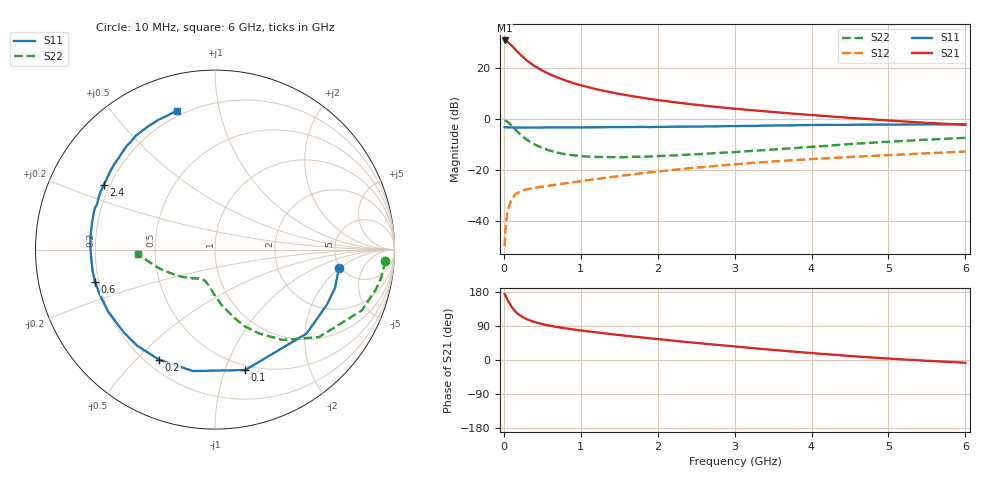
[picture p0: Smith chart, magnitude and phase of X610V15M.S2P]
! SIEMENS Small Signal Semiconductors
! BFP193W
! Si NPN RF Bipolar Junction Transistor in SOT343
! VCE = 10 V  IC = 15 mA
! Common Emitter S-Parameters:  April 1994
# GHz  S  MA  R  50
!  f  S11  S21  S12  S22
! GHz  MAG  ANG  MAG  ANG  MAG  ANG  MAG  ANG
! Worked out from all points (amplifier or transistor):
!   40 points, 10 MHz to 6 GHz, reference 50 ohm
!   highest |S21| = 31.0 dB at 10 MHz (marker M1)
!   |S21| within 3 dB of that: start of sweep to 132.5 MHz
!   unconditionally stable (mu >= 1): 1.187 GHz to 4.775 GHz
!   at 200 MHz: K = 0.28, MSG = 27.2 dB, |S12| = -28.6 dB
!   at 1.5 GHz: K = 1.07, MAG = 14.5 dB, |S12| = -22.3 dB
!   at 6 GHz: K = 0.93, MSG = 5.2 dB, |S12| = -12.7 dB
!   S11 on the Smith chart (normalised r, x): 10 MHz: 4.83, -1.92; 100 MHz: 0.46, -1.18; 200 MHz: 0.25, -0.59; 600 MHz: 0.19, -0.13; 2.4 GHz: 0.18, +0.26; 6 GHz: 0.17, +0.75
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0.01  0.698 -8.4  35.51 174.1  0.0032 77.6  0.9509 -3.8
0.02  0.7016 -17.6  35.29 170.6  0.0067 77.1  0.94 -9.4
0.03  0.6952 -26.1  34.82 166.3  0.0098 76.1  0.9242 -13.8
0.05  0.6922 -42.5  33.37 157.9  0.0157 68.8  0.8859 -22.5
0.1  0.6919 -75.9  28.39 140.7  0.0266 56.2  0.7573 -40.0
0.15  0.6877 -100.3  23.55 127.8  0.0335 47.2  0.6296 -53.1
0.2  0.6881 -116.9  19.59 119.0  0.0372 41.9  0.5286 -62.2
0.25  0.6892 -128.9  16.63 112.6  0.0402 38.9  0.4553 -69.1
0.3  0.6866 -137.5  14.28 107.5  0.0419 37.0  0.395 -74.2
0.4  0.6887 -150.0  11.12 100.1  0.0449 35.5  0.32 -82.1
0.5  0.6894 -158.7  9.079 94.7  0.0474 36.1  0.273 -87.8
0.6  0.6921 -164.8  7.633 90.4  0.0499 36.9  0.2416 -92.3
0.8  0.6908 -173.9  5.802 83.6  0.0552 39.8  0.2065 -98.8
1.1  0.6954 176.8  4.272 75.4  0.0638 43.3  0.1841 -106.4
1.3  0.6983 171.5  3.623 70.4  0.0701 45.2  0.1809 -110.3
1.6  0.7034 164.8  2.972 63.6  0.08 47.2  0.1807 -114.9
2.2  0.7141 153.3  2.186 51.1  0.1012 48.3  0.1942 -124.5
2.4  0.7175 149.8  2.005 47.1  0.1082 48.2  0.2022 -127.3
3.2  0.7408 136.4  1.521 32.1  0.1375 46.0  0.2378 -140.3
4.5  0.7805 118.9  1.067 10.5  0.1816 39.6  0.3261 -161.0
5.5  0.7921 109.8  0.851 -2.0  0.2146 34.4  0.3975 -172.7
6  0.8024 105.5  0.777 -7.3  0.2323 32.1  0.4321 -177.1
